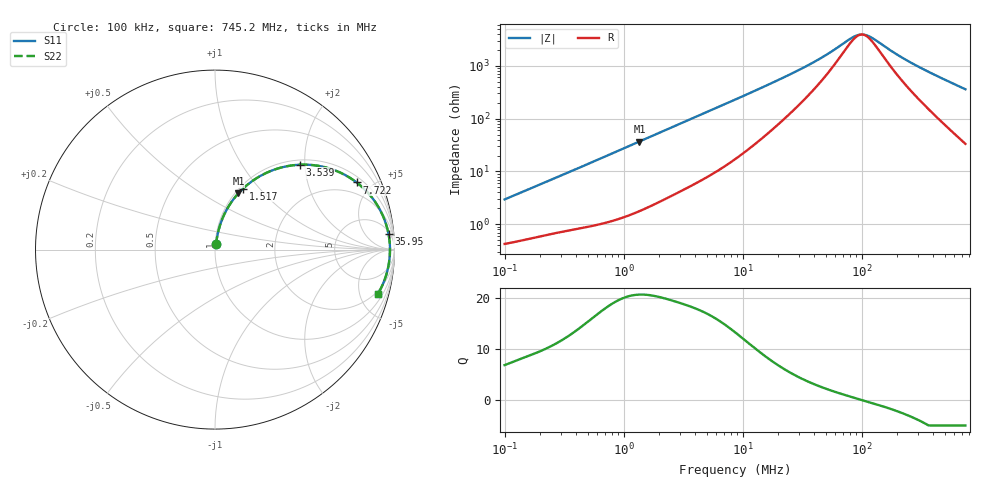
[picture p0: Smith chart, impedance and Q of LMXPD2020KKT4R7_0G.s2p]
! LMXPD2020KKT4R7_0G  S-PARAMETER MODEL  ( General Type )
! Model Generated by TAIYO YUDEN Corporation (https://www.yuden.co.jp/en/)
! Version 1.0
! TAIYO YUDEN Control No. 191023NI43SB-FBB
! Copyright(c) 2019 TAIYO YUDEN CO.,LTD. All Rights Reserved.
! Product Description (link to TY-COMPAS)
! https://ds.yuden.co.jp/TYCOMPAS/or/detail?pn=LMXPD2020KKT4R7M0G&u=M
! Products Name : Inductors
! Characteristics :
!  Inductance : 4.7 uH , SRF(min) : -Hz , DC Resistance(max) : 0.384 Ohm
!  Rated Current : Saturation :760 mA , Temp Rise : 820 mA (40 degC)
!  Case Size : 2.0 x 2.0 / 0.079 x 0.079 [mm/inch] , Thickness : 1 / 0.039 [mm/inch]
!  (Conditions: Temperature = 25 degC , DC Bias Current/Voltage = 0A / 0V)
! External Node Assignments :
!  1  o---GGG---o  2
! GND o---------o GND
! Frequency Range : 0.1MHz  -  745.243127MHz  [ 402 STEP ]
# MHz S RI R 50
! Freq[MHz].  S11 Real  S11 Imag  S21 Real  S21 Imag  S12 Real  S12 Imag  S22 Real  S22 Imag
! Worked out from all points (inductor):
!   401 points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, 100 kHz to 745.2 MHz, reference 50 ohm
!   read as one part in series: L = 4.62 uH near 104.6 kHz
!   highest Q = 20.7 at 1.357 MHz (marker M1), where L = 4.31 uH
!   self-resonance near 100.5 MHz
!   S11 on the Smith chart (normalised r, x): 100 kHz: 1.01, +0.06; 1.517 MHz: 1.04, +0.82; 3.539 MHz: 1.10, +1.88; 7.722 MHz: 1.29, +4.06; 35.95 MHz: 7, +20; 745.2 MHz: 1.67, -7.15
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0.1  0.00508 0.029  0.9949 -0.029  0.9949 -0.029  0.00508 0.029
0.228133  0.0104 0.0636  0.9896 -0.0636  0.9896 -0.0636  0.0104 0.0636
0.445256  0.023 0.1193  0.977 -0.1193  0.977 -0.1193  0.023 0.1193
0.831133  0.059 0.211  0.941 -0.211  0.941 -0.211  0.059 0.211
1.35721  0.1308 0.314  0.8692 -0.314  0.8692 -0.314  0.1308 0.314
1.517228  0.1559 0.3395  0.8441 -0.3395  0.8441 -0.3395  0.1559 0.3395
1.98253  0.2326 0.3986  0.7674 -0.3986  0.7674 -0.3986  0.2326 0.3986
3.539315  0.4711 0.4729  0.5289 -0.4729  0.5289 -0.4729  0.4711 0.4729
5.056047  0.6334 0.4533  0.3666 -0.4533  0.3666 -0.4533  0.6334 0.4533
7.722275  0.7893 0.3741  0.2107 -0.3741  0.2107 -0.3741  0.7893 0.3741
8.632747  0.8204 0.3482  0.1796 -0.3482  0.1796 -0.3482  0.8204 0.3482
15.75902  0.9239 0.2127  0.0761 -0.2127  0.0761 -0.2127  0.9239 0.2127
35.95147  0.9667 0.0875  0.0333 -0.0875  0.0333 -0.0875  0.9667 0.0875
38.43783  0.968 0.0802  0.032 -0.0802  0.032 -0.0802  0.968 0.0802
53.69948  0.9725 0.0483  0.0275 -0.0483  0.0275 -0.0483  0.9725 0.0483
82.01707  0.9748 0.0148  0.0252 -0.0148  0.0252 -0.0148  0.9748 0.0148
95.86707  0.975 0.00345  0.025 -0.00345  0.025 -0.00345  0.975 0.00345
104.8075  0.975 -0.00301  0.025 0.00301  0.025 0.00301  0.975 -0.00301
117.1645  0.9749 -0.0111  0.0251 0.0111  0.0251 0.0111  0.9749 -0.0111
171.1468  0.9734 -0.0403  0.0266 0.0403  0.0266 0.0403  0.9734 -0.0403
319.4697  0.9641 -0.1025  0.0359 0.1025  0.0359 0.1025  0.9641 -0.1025
745.2431  0.9085 -0.2455  0.0915 0.2455  0.0915 0.2455  0.9085 -0.2455
